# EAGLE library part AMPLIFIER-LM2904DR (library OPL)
DUAL OPERATIONAL AMPLIFIERS
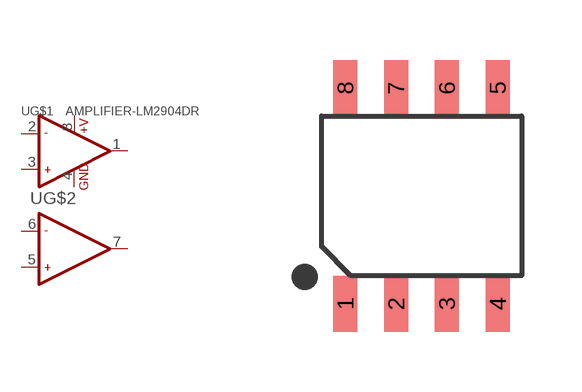
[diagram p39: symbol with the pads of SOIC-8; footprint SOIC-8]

Designator prefix U; gates G$1=OPAMP_2-1 G$2=OPAMP_2_1-1

## AMPLIFIER-LM2904DR-310020015  [SOIC-8]
1  G$1:OUT1  out
2  G$1:-IN1  in
3  G$1:+IN1  in
4  G$1:GND  pwr
5  G$2:+IN2  in
6  G$2:-IN2  in
7  G$2:OUT2  out
8  G$1:+V  pwr

## Footprint SOIC-8 (pad centres in mm)
smd 0.6 x 1.4: 1 -1.905,-2.7; 2 -0.635,-2.7; 3 0.635,-2.7; 4 1.905,-2.7; 5 1.905,2.7; 6 0.635,2.7; 7 -0.635,2.7; 8 -1.905,2.7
